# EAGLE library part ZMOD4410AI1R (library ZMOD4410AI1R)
The ZMOD4410 gas sensor module is an easily integrated firmware configurable architecture enabling multiple sensing solutions with a common hardware platform. Simply download one of the firmware libraries that best supports your application from the Renesas website and integrate it with your host microcontroller. The JEDEC JESD47 qualified device supports 10+ years of life, supporting your indoor air quality (IAQ) application designed for detecting total volatile organic compounds (TVOCs), estimating CO2, a Source: Datasheet
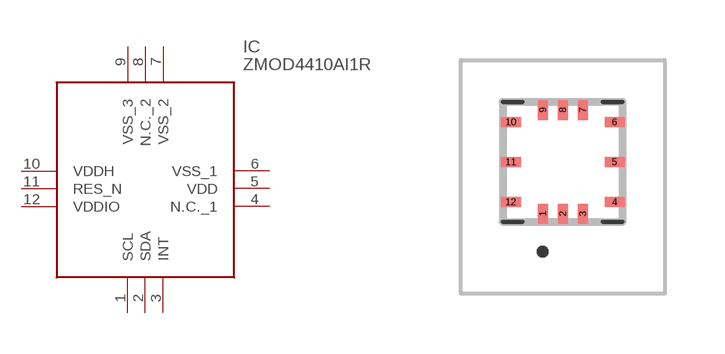
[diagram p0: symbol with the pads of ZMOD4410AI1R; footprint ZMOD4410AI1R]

Designator prefix IC

## ZMOD4410AI1R (Description: The ZMOD4410 gas sensor module is an easily integrated firmware configurable architecture enabling multiple sensing solutions with a common hardware platform. Simply download one of the firmware libraries that best supports your application from the Renesas website and integrate it with your host microcontroller. The JEDEC JESD47 qualified device supports 10+ years of life, supporting your indoor air quality (IAQ) application designed for detecting total volatile organic compounds (TVOCs), estimating CO2, a; Height: 0.77mm; Manufacturer_Name: Renesas Electronics; Manufacturer_Part_Number: ZMOD4410AI1R; Mouser_Part_Number: 964-ZMOD4410AI1R; Mouser_Price-Stock: https://www.mouser.co.uk/ProductDetail/Renesas-Electronics/ZMOD4410AI1R?qs=y6ZabgHbY%252BwCtZi1inoY6g%3D%3D)  [ZMOD4410AI1R]
1  SCL
2  SDA
3  INT
4  N.C._1
5  VDD
6  VSS_1
7  VSS_2
8  N.C._2
9  VSS_3
10  VDDH
11  RES_N
12  VDDIO

## Footprint ZMOD4410AI1R (pad centres in mm)
LGG12D1
smd 0.25 x 0.5: 1 -0.5,-1.3; 2 0,-1.3; 3 0.5,-1.3; 7 0.5,1.3; 8 0,1.3; 9 -0.5,1.3
smd 0.5 x 0.25: 4 1.3,-1; 5 1.3,0; 6 1.3,1; 10 -1.3,1; 11 -1.3,0; 12 -1.3,-1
